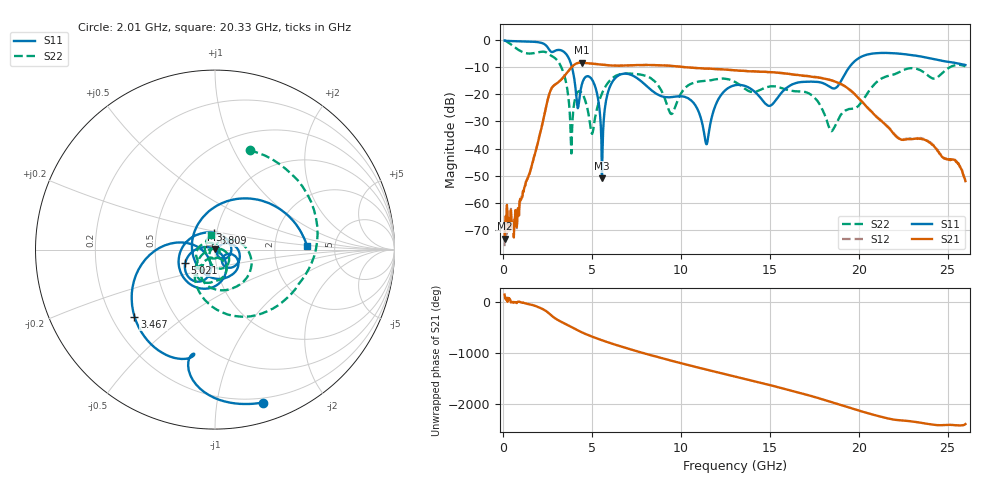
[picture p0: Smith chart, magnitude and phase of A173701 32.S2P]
!  2-Port S-parameters saved by WinCal
! VAR MeasName=S-Parameters (CALIBRATED_DATA) read from VNA (N5245A)
! VAR MeasDate=2017-6-7 10:30:29
! VAR NAME=A173701 32
! VAR FILENAME=A173701 32.S2P
! VAR DATE=2017-6-7 10:30:29
! VAR PHYS_PORTS=1,2
# Hz S DB R 50
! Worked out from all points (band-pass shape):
!   801 points, 100 MHz to 26 GHz, reference 50 ohm
!   highest |S21| = -8.46 dB at 4.438 GHz (marker M1); lowest = -73.1 dB at 100 MHz (marker M2)
!   |S21| within 3 dB of the highest: 3.689 GHz to 13.45 GHz (9.759 GHz wide, 114 % of centre)
!   lowest |S11| = -50.9 dB at 5.571 GHz (marker M3), VSWR 1.01, Z = 49.8 + j0.232 ohm
!   |S11| at or under -10 dB: 3.879 GHz to 19.49 GHz (15.61 GHz wide, 134 % of centre)
!   |S22| runs from -41.8 to -0.3 dB; largest |S21 - S12| = 0.004
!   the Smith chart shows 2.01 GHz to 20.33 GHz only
!   S11 on the Smith chart (normalised r, x): 2.01 GHz: 0.16, -1.35; 3.467 GHz: 0.29, -0.33; 5.021 GHz: 0.71, -0.11; 8.809 GHz: 0.97, +0.18; 20.33 GHz: 3.10, +0.16
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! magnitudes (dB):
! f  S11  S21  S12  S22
! 100 MHz  -0.3  -73.1  -75.8  -0.3
! 682.8 MHz  -0.6  -65.4  -64.3  -2.9
! 2.01 GHz  -1.0  -36.8  -36.7  -4.6
! 3.467 GHz  -4.7  -13.3  -13.3  -13.4
! 3.856 GHz  -9.4  -10.2  -10.2  -41.8
! 4.212 GHz  -25.2  -8.6  -8.6  -19.2
! 4.438 GHz  -16.6  -8.5  -8.5  -19.6
! 5.021 GHz  -14.8  -8.8  -8.8  -34.6
! 5.571 GHz  -50.9  -9.1  -9.2  -19.8
! 6.478 GHz  -13.3  -9.6  -9.5  -12.9
! 8.744 GHz  -20.3  -9.4  -9.4  -17.0
! 8.809 GHz  -20.5  -9.4  -9.4  -17.6
! 9.489 GHz  -21.1  -9.7  -9.7  -27.3
! 10.72 GHz  -23.2  -10.4  -10.4  -15.9
! 11.43 GHz  -38.3  -10.6  -10.6  -15.1
! 13.05 GHz  -16.7  -11.3  -11.3  -15.5
! 14.99 GHz  -24.3  -11.9  -11.9  -17.2
! 17.39 GHz  -15.4  -13.7  -13.5  -20.5
! 18.49 GHz  -17.7  -15.0  -15.0  -33.6
! 20.33 GHz  -5.8  -23.8  -23.8  -21.3
! 21.69 GHz  -4.9  -32.4  -32.3  -13.3
! 26 GHz  -9.3  -51.9  -52.2  -9.9
